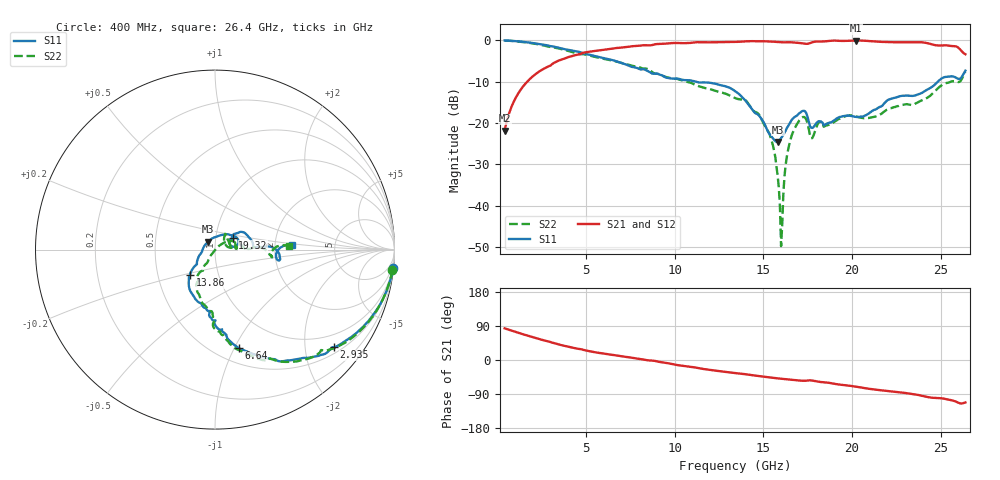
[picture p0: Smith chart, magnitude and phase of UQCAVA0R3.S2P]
!  Part Number  UQCAVA0R3
!  Description: RF capacitor  Mounting Orientation: Horizontal
!  Application:
# GHZ S DB R 50
! Freq  |S11|  S11 Ph  |S21|  S21 Ph  |S12|  S12 Ph  |S22|  S22 Ph
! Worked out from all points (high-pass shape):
!   401 points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, 400 MHz to 26.4 GHz, reference 50 ohm
!   highest |S21| = -0.04 dB at 20.23 GHz (marker M1); lowest = -21.9 dB at 400 MHz (marker M2)
!   |S21| within 3 dB of the highest: 4.801 GHz to 26.29 GHz (21.49 GHz wide, 138 % of centre)
!   lowest |S11| = -24.6 dB at 15.8 GHz (marker M3), VSWR 1.12, Z = 46.2 + j4.18 ohm
!   |S11| at or under -10 dB: 11.2 GHz to 24.84 GHz (13.65 GHz wide, 75.7 % of centre)
!   |S22| runs from -49.9 to 0.0 dB; largest |S21 - S12| = 0.0033
!   S11 on the Smith chart (normalised r, x): 400 MHz: 0, -19; 2.935 GHz: 0.65, -2.66; 6.64 GHz: 0.65, -1.04; 13.86 GHz: 0.73, -0.22; 19.32 GHz: 1.21, +0.16; 26.4 GHz: 2.50, +0.16
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0.4  -0.02 -5.9  -21.88 83.5  -21.89 83.5  -0.05 -6.6
1.375  -0.32 -19.8  -11.54 68.9  -11.54 68.9  -0.37 -21.9
2.935  -1.33 -39.3  -6.18 48.1  -6.19 48.2  -1.55 -42.3
4.755  -3.05 -61.0  -3.11 28.1  -3.11 28.1  -3.35 -63.4
6.64  -4.97 -76.6  -1.90 12.4  -1.90 12.4  -5.04 -78.6
9.11  -8.23 -92.6  -0.87 -4.8  -0.87 -4.8  -8.21 -91.4
13.4  -12.28 -127.0  -0.37 -34.4  -0.37 -34.4  -13.96 -118.5
13.855  -14.00 -134.6  -0.27 -36.6  -0.26 -36.7  -14.30 -118.0
15.285  -22.28 -167.7  -0.25 -45.7  -0.24 -45.8  -22.16 -120.8
15.61  -24.09 160.0  -0.34 -47.6  -0.34 -47.6  -26.78 -125.5
15.805  -24.61 130.0  -0.39 -48.5  -0.39 -48.5  -32.78 -122.5
16  -23.68 100.3  -0.44 -49.3  -0.44 -49.4  -49.85 -97.7
16.13  -22.88 84.7  -0.47 -49.7  -0.46 -49.8  -36.89 44.3
16.325  -21.26 68.5  -0.45 -50.5  -0.46 -50.6  -28.16 41.2
16.715  -18.76 45.8  -0.50 -52.7  -0.50 -52.8  -21.83 32.9
17.3  -17.06 21.4  -0.77 -54.9  -0.77 -55.0  -18.56 15.9
17.755  -21.21 23.8  -0.46 -54.3  -0.45 -54.3  -23.70 33.4
19.315  -18.55 33.0  -0.12 -65.0  -0.12 -65.0  -18.95 10.1
20.225  -18.54 31.8  -0.04 -70.4  -0.04 -70.5  -18.45 2.1
22.11  -14.29 26.9  -0.45 -82.1  -0.44 -82.2  -16.51 9.5
23.995  -12.59 3.7  -0.49 -95.0  -0.49 -95.1  -14.44 1.0
26.4  -7.33 3.5  -3.36 -112.0  -3.35 -112.1  -7.64 2.8
